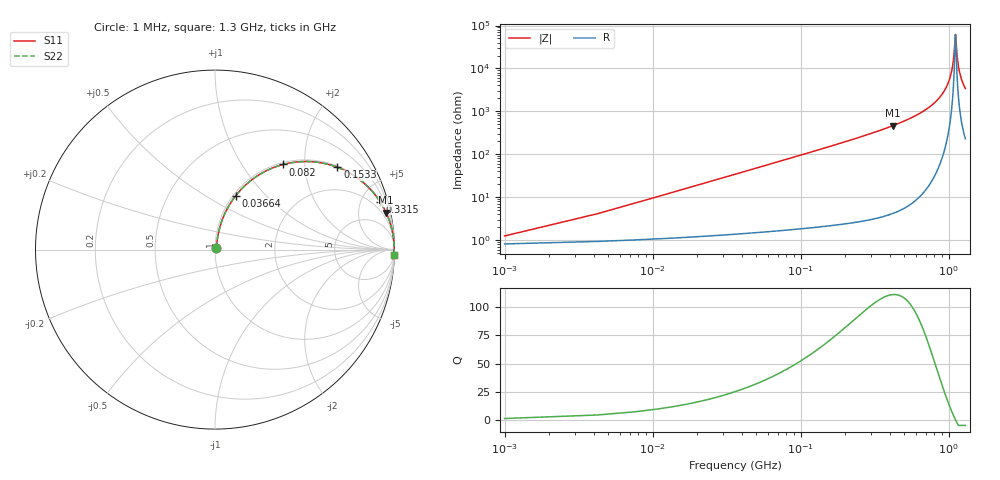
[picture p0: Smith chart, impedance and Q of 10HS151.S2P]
! Coilcraft 1008HS-151 Chip Inductor
! 02 July 2002
# MHZ S MA R 50
!Freq  MagS11  AngS11  MagS21  AngS21  MagS12  AngS12  MagS22  AngS22
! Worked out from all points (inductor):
!   402 points, 1 MHz to 1.3 GHz, reference 50 ohm
!   read as one part in series: L = 150 nH near 7.48 MHz
!   highest Q = 111 at 422.2 MHz (marker M1), where L = 175 nH
!   self-resonance near 1.112 GHz
!   S11 on the Smith chart (normalised r, x): 1 MHz: 1.02, +0.02; 36.64 MHz: 1.03, +0.69; 82 MHz: 1.03, +1.55; 153.3 MHz: 1.04, +2.94; 331.5 MHz: 1.06, +6.85; 1.3 GHz: 6, -68
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1  0.01233 48.8  0.9919 -0.5  0.9919 -0.5  0.01233 48.8
10.72  0.1 78.3  0.9846 -5.7  0.9846 -5.7  0.1 78.3
13.96  0.1295 77.8  0.9807 -7.4  0.9807 -7.4  0.1295 77.8
23.68  0.2157 74.4  0.9646 -12.4  0.9646 -12.4  0.2157 74.4
36.64  0.323 68.9  0.9337 -18.8  0.9337 -18.8  0.323 68.9
82  0.6072 51.4  0.7813 -37.4  0.7813 -37.4  0.6072 51.4
153.28  0.8218 33.9  0.5581 -55.3  0.5581 -55.3  0.8218 33.9
218.08  0.9018 25.0  0.4219 -64.4  0.4219 -64.4  0.9018 25.0
331.48  0.9575 16.2  0.2794 -73.2  0.2794 -73.2  0.9575 16.2
422.2  0.9758 12.1  0.21 -77.4  0.21 -77.4  0.9758 12.1
435.16  0.9776 11.7  0.202 -77.8  0.202 -77.8  0.9776 11.7
652.24  0.9931 6.1  0.1062 -83.2  0.1062 -83.2  0.9931 6.1
869.32  0.9976 2.7  0.04768 -85.7  0.04768 -85.7  0.9976 2.7
1011.88  0.9984 1.1  0.01843 -84.5  0.01843 -84.5  0.9984 1.1
1057.24  0.9984 0.6  0.01013 -80.9  0.01013 -80.9  0.9984 0.6
1086.4  0.9984 0.3  0.00508 -72.0  0.00508 -72.0  0.9984 0.3
1109.08  0.9984 0.1  0.001832 -29.7  0.001832 -29.7  0.9984 0.1
1115.56  0.9984 -0.0  0.001614 7.0  0.001614 7.0  0.9984 -0.0
1144.72  0.9983 -0.3  0.005365 71.7  0.005365 71.7  0.9983 -0.3
1177.12  0.9982 -0.6  0.01055 80.0  0.01055 80.0  0.9982 -0.6
1228.96  0.998 -1.1  0.01871 83.3  0.01871 83.3  0.998 -1.1
1300  0.9976 -1.7  0.02944 84.4  0.02944 84.4  0.9976 -1.7
